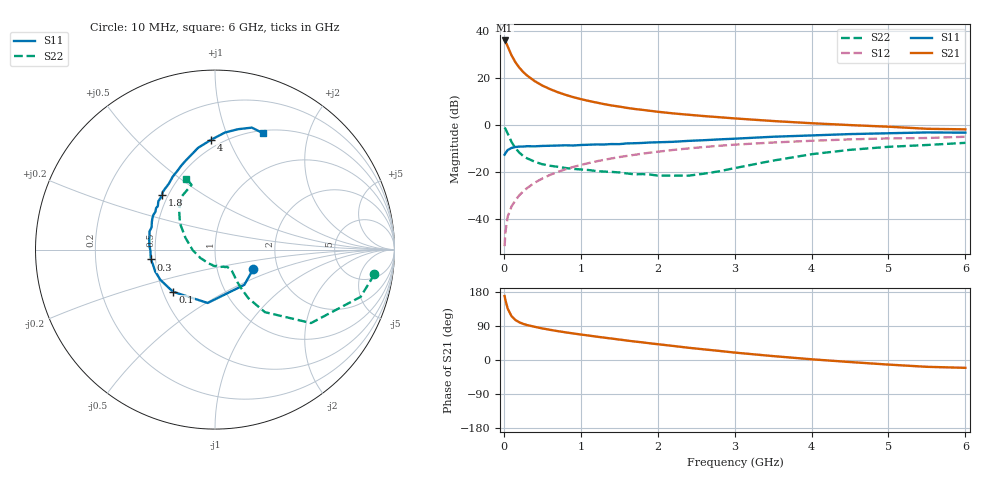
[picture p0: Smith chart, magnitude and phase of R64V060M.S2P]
! SIEMENS Small Signal Semiconductors
! BFR193
! Si NPN RF Bipolar Junction Transistor in SOT23
! VCE = 4 V  IC = 60 mA
! Common Emitter S-Parameters:  May  1996
# GHz  S  MA  R  50
!  f  S11  S21  S12  S22
! GHz  MAG  ANG  MAG  ANG  MAG  ANG  MAG  ANG
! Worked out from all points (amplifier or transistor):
!   36 points, 10 MHz to 6 GHz, reference 50 ohm
!   highest |S21| = 36.2 dB at 10 MHz (marker M1)
!   |S21| within 3 dB of that: start of sweep to 56.37 MHz
!   unconditionally stable (mu >= 1): 356.6 MHz to 1.874 GHz; 1.989 GHz to 2.005 GHz
!   at 250 MHz: K = 0.97, MSG = 25.4 dB, |S12| = -28.1 dB
!   at 1.4 GHz: K = 1.02, MAG = 10.4 dB, |S12| = -14.1 dB
!   at 6 GHz: K = 0.95, MSG = 1.6 dB, |S12| = -4.8 dB
!   S11 on the Smith chart (normalised r, x): 10 MHz: 1.50, -0.34; 100 MHz: 0.56, -0.30; 300 MHz: 0.47, -0.06; 1.8 GHz: 0.46, +0.34; 4 GHz: 0.44, +0.87; 6 GHz: 0.53, +1.35
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0.01  0.2392 -26.8  64.32 168.9  0.0027 78.1  0.8992 -8.8
0.02  0.2554 -50.2  61.39 158.6  0.0053 76.0  0.8527 -18.0
0.05  0.3002 -97.8  48.16 135.6  0.0115 70.4  0.6738 -37.4
0.1  0.3318 -135.0  31.06 115.7  0.0189 70.6  0.446 -51.4
0.15  0.3479 -151.0  22.15 105.5  0.0255 71.5  0.3288 -55.5
0.2  0.3548 -160.0  17.08 99.6  0.0326 73.2  0.2659 -55.9
0.25  0.3557 -166.7  13.78 95.4  0.0393 73.6  0.2251 -55.5
0.3  0.3616 -171.3  11.6 92.3  0.0462 74.9  0.2006 -54.7
0.4  0.3597 -178.7  8.804 87.6  0.0604 74.9  0.1696 -52.9
0.5  0.3666 176.1  7.066 83.4  0.0742 75.0  0.1496 -51.6
0.6  0.37 172.0  5.933 79.7  0.0887 74.2  0.1389 -51.7
0.7  0.3733 168.0  5.109 76.2  0.1024 73.2  0.1319 -52.5
0.8  0.3788 164.5  4.49 73.1  0.1166 71.8  0.1246 -53.7
1.1  0.3889 154.0  3.334 64.6  0.158 68.1  0.1126 -60.0
1.4  0.4018 144.8  2.663 56.6  0.1983 63.8  0.1028 -69.4
1.8  0.4245 134.1  2.148 46.6  0.2509 57.7  0.0923 -88.3
2.2  0.4485 124.9  1.806 37.1  0.3007 51.6  0.0856 -116.9
3.5  0.575 99.4  1.242 10.3  0.4336 31.0  0.1787 157.8
4  0.6131 91.9  1.115 1.9  0.4716 23.9  0.2442 143.1
4.5  0.6548 85.1  1.018 -5.4  0.5052 16.9  0.3028 131.4
5.5  0.7099 73.2  0.849 -18.0  0.5406 3.2  0.3838 109.9
6  0.7019 67.7  0.826 -20.7  0.5747 -0.8  0.4264 112.0
